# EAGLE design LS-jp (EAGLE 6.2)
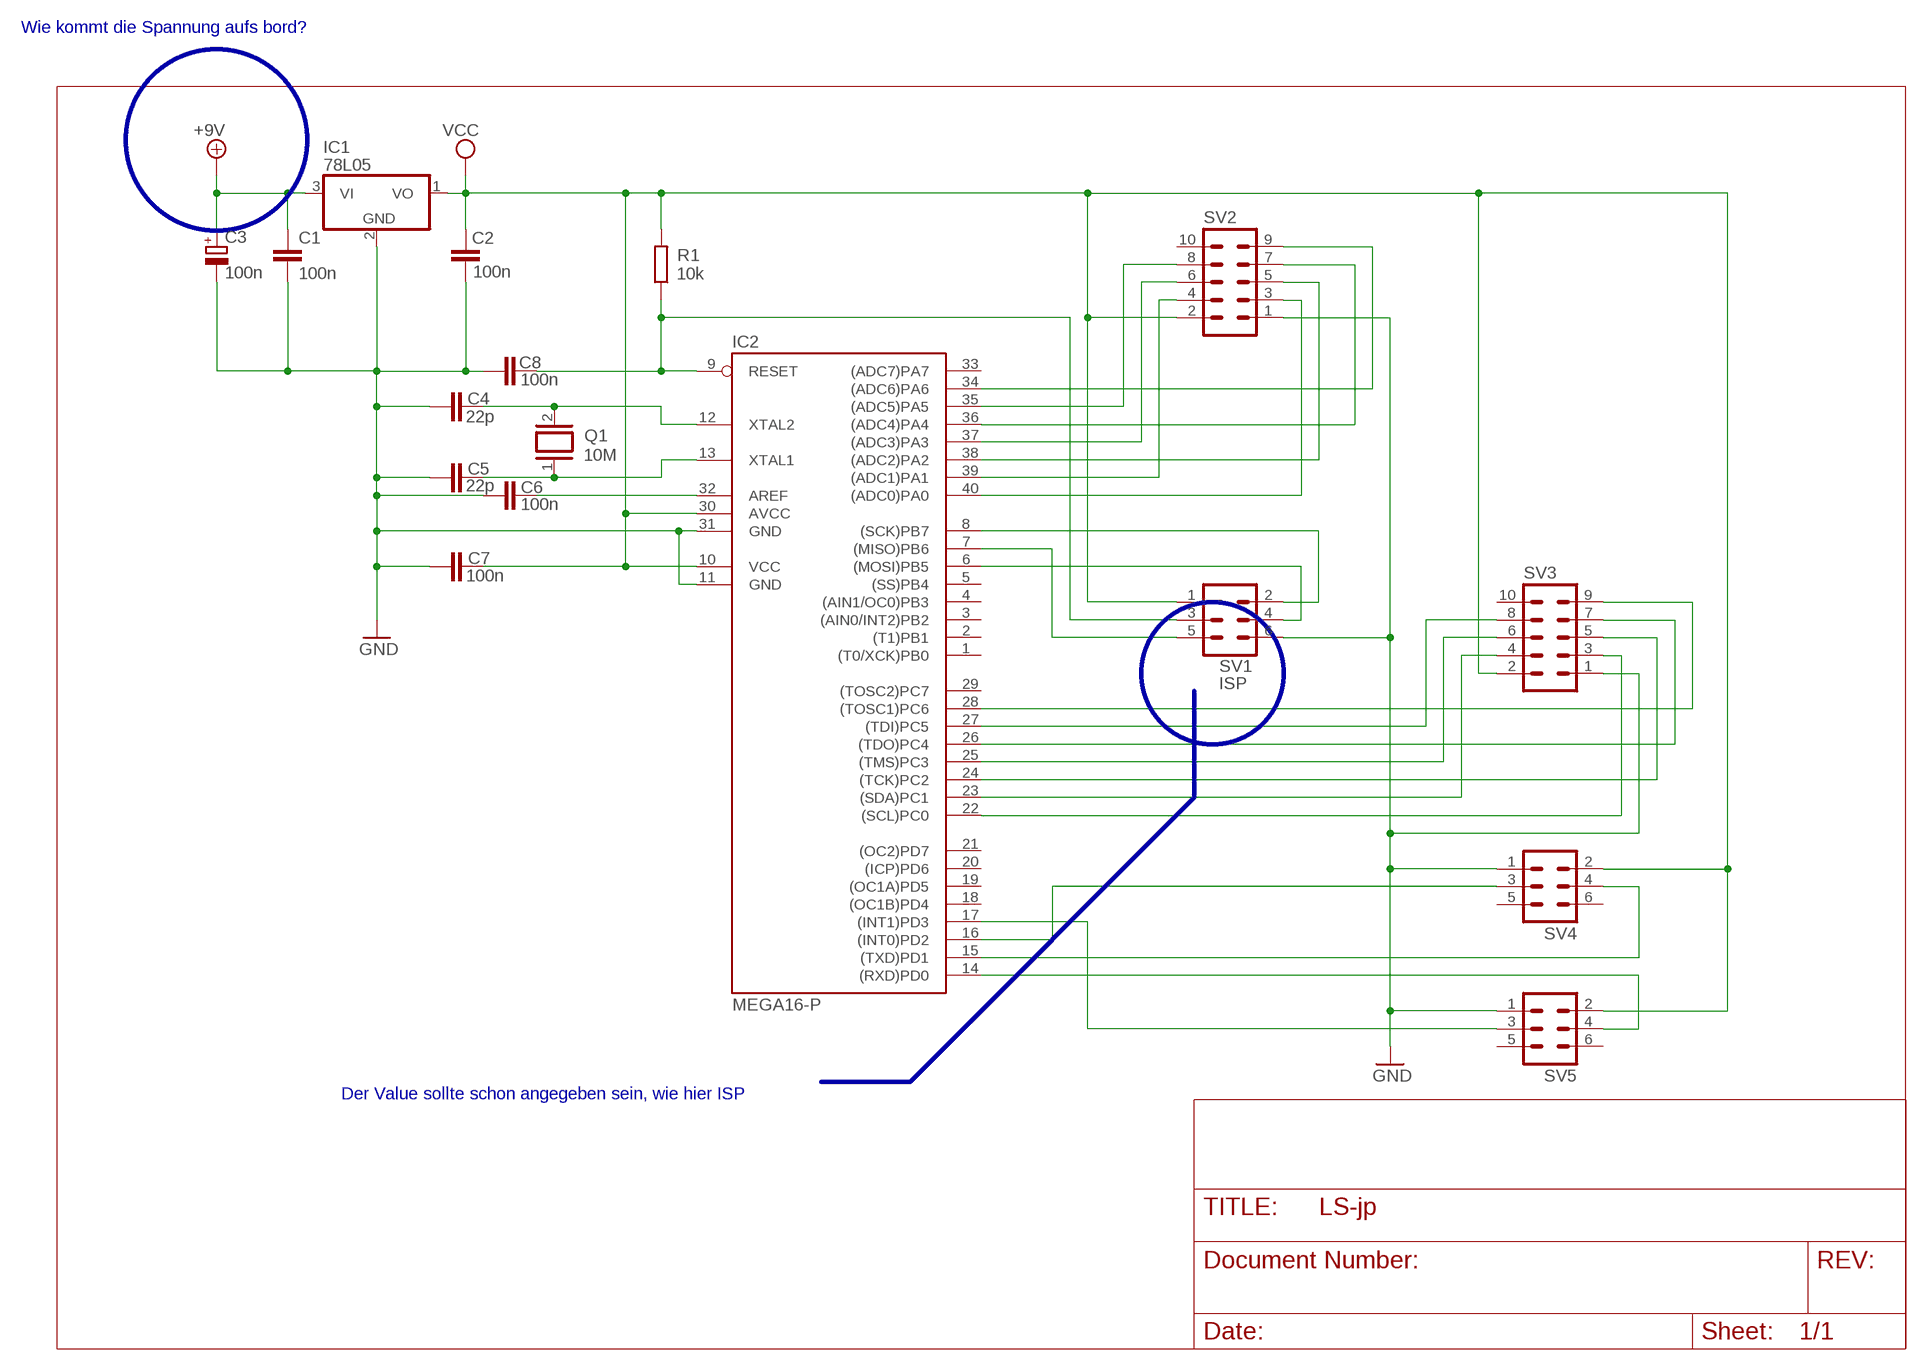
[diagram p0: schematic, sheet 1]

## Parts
C1  100n  C-EU025-024X044  [C025-024X044]
C2  100n  C-EU025-024X044  [C025-024X044]
C3  100n  CPOL-EUE2.5-7  [E2,5-7]
C4  22p  C-EU025-024X044  [C025-024X044]
C5  22p  C-EU025-024X044  [C025-024X044]
C6  100n  C-EU025-024X044  [C025-024X044]
C7  100n  C-EU025-024X044  [C025-024X044]
C8  100n  C-EU025-024X044  [C025-024X044]
IC1  78L05  78L12Z  [TO92]
IC2  MEGA16-P  [DIL40]
Q1  10M  XTAL/S  [QS]
R1  10k  R-EU_0207/10  [0207/10]
SV1  ISP  ML6  [ML6]
SV2  ML10  [ML10]
SV3  ML10  [ML10]
SV4  ML6  [ML6]
SV5  ML6  [ML6]

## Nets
+9V: C1.1 C3.+ IC1.3(VI)
GND: C1.2 C2.2 C3.- C4.2 C5.2 C6.2 C7.1 C8.1 IC1.2(GND) IC2.11(GND) IC2.31(GND) SV1.6 SV2.1 SV3.1 SV4.1 SV5.1
N$1: C6.1 IC2.32(AREF)
N$2: IC2.22((SCL)PC0) SV3.3
N$3: IC2.23((SDA)PC1) SV3.4
N$4: C8.2 IC2.9(RESET) R1.1 SV1.3
N$5: IC2.24((TCK)PC2) SV3.5
N$6: IC2.7((MISO)PB6) SV1.5
N$7: IC2.6((MOSI)PB5) SV1.4
N$8: C4.1 IC2.12(XTAL2) Q1.2
N$9: C5.1 IC2.13(XTAL1) Q1.1
N$10: IC2.8((SCK)PB7) SV1.2
N$11: IC2.40((ADC0)PA0) SV2.3
N$13: IC2.39((ADC1)PA1) SV2.4
N$14: IC2.25((TMS)PC3) SV3.6
N$15: IC2.38((ADC2)PA2) SV2.5
N$16: IC2.37((ADC3)PA3) SV2.6
N$17: IC2.36((ADC4)PA4) SV2.7
N$18: IC2.35((ADC5)PA5) SV2.8
N$19: IC2.26((TDO)PC4) SV3.7
N$20: IC2.27((TDI)PC5) SV3.8
N$21: IC2.28((TOSC1)PC6) SV3.9
N$22: IC2.34((ADC6)PA6) SV2.9
N$23: IC2.15((TXD)PD1) SV4.4
N$24: IC2.14((RXD)PD0) SV5.4
N$25: IC2.16((INT0)PD2) SV4.3
N$26: IC2.17((INT1)PD3) SV5.3
VCC: C2.1 C7.2 IC1.1(VO) IC2.10(VCC) IC2.30(AVCC) R1.2 SV1.1 SV2.2 SV3.2 SV4.2 SV5.2
Unconnected: IC2.1((T0/XCK)PB0) IC2.2((T1)PB1) IC2.3((AIN0/INT2)PB2) IC2.4((AIN1/OC0)PB3) IC2.5((SS)PB4) IC2.18((OC1B)PD4) IC2.19((OC1A)PD5) IC2.20((ICP)PD6) IC2.21((OC2)PD7) IC2.29((TOSC2)PC7) IC2.33((ADC7)PA7) SV2.10 SV3.10 SV4.5 SV4.6 SV5.5 SV5.6

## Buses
B$1

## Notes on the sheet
- Wie kommt die Spannung aufs bord?
- Der Value sollte schon angegeben sein, wie hier ISP

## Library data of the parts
C1 C2 C4-C8 = rcl:C-EU: CAPACITOR, European symbol
C3 = rcl:CPOL-EU: POLARIZED CAPACITOR, European symbol
IC1 = linear:78*: Positive VOLTAGE REGULATOR Source: http://cache.national.com/ds/LM/LM78L05.pdf http://www.fairchildsemi.com/ds/LM/LM7805.pdf
IC2 = atmel:MEGA16-P: MICROCONTROLLER 16 Kbytes FLASH 1 kbytes SRAM 512 bytes EEPROM USART 8-channel 10 bit ADC Source: avr.lbr; MPN: ATMEGA16-16PU; OC_FARNELL: 9171142; OC_NEWARK: 01M6885
Q1 = special:XTAL/S: CRYSTAL
R1 = rcl:R-EU_: RESISTOR, European symbol
SV1 SV4 SV5 = con-harting-ml:ML6: HARTING; OC_FARNELL: unknown; OC_NEWARK: unknown
SV2 SV3 = con-harting-ml:ML10: HARTING; OC_FARNELL: unknown; OC_NEWARK: unknown

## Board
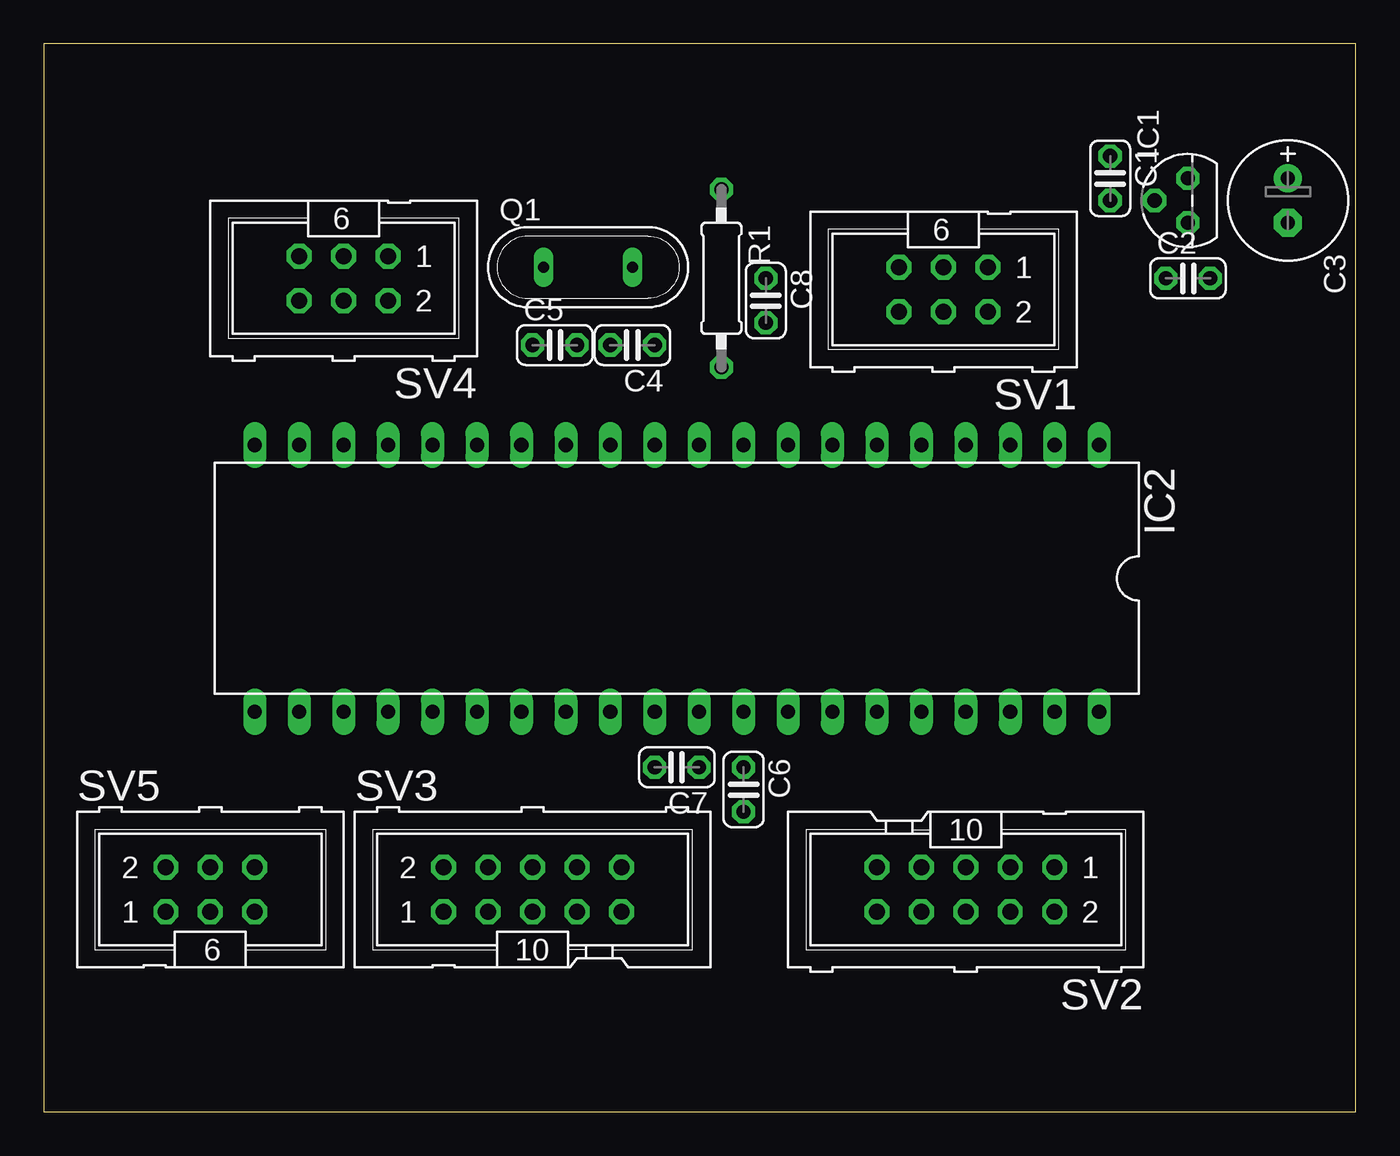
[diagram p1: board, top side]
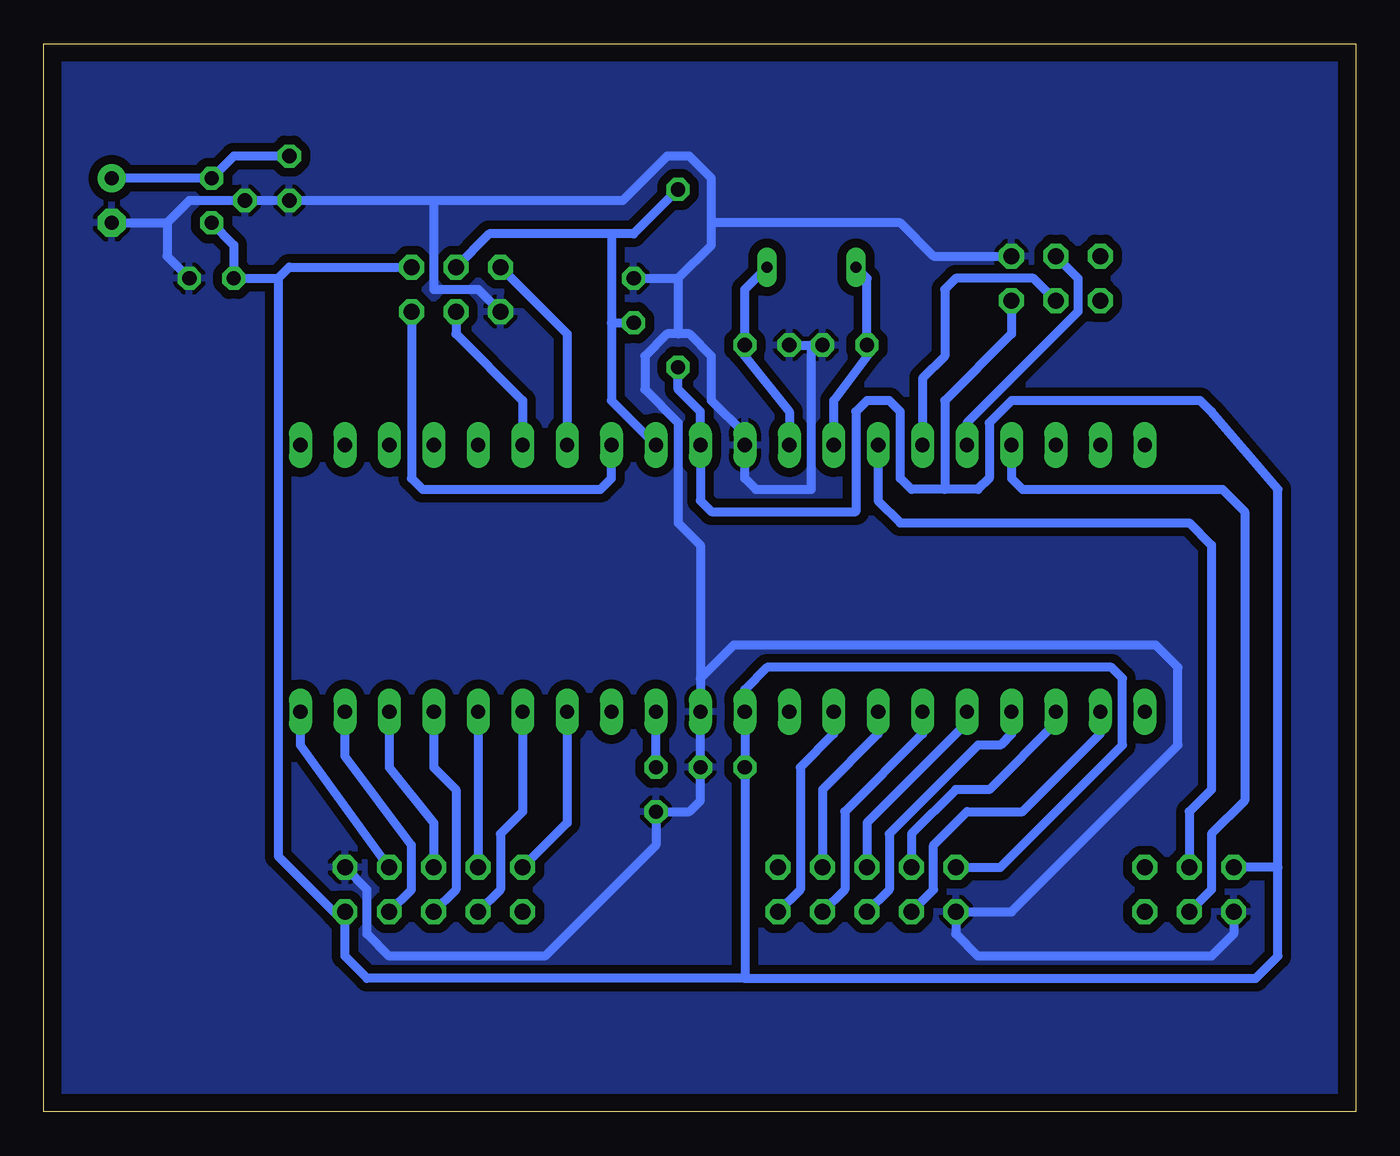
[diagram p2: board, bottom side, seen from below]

Size 75 x 61.03 mm. Coordinates in mm from the lower left corner, seen from the top.
Outline: 0,0 75,0 75,61.03 0,61.03 0,0
Copper layers (1*16): Top 0.035mm / dielectric 1.5mm / Bottom 0.035mm
Design rules "default": minimum track width 10mil, minimum drill 24mil, track to track 8mil, track to pad 8mil, pad to pad 8mil, via to via 8mil, smd to smd 8mil, copper to edge 40mil, drill to drill 8mil, minimum pad ring 10mil, minimum via ring 8mil, stop-mask expansion 4mil, vias tented up to drill 0mil, thermal gap 10mil

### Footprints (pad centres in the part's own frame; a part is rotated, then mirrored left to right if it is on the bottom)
C025-024X044 = drill 0.813 octagon: 1 -1.27,0; 2 1.27,0
E2,5-7 = drill 0.813 pad 1.6: + -1.27,0 | drill 0.813 pad 1.6 octagon: - 1.27,0
TO92 = drill 0.813 octagon: 1 -1.27,0; 2 0,1.905; 3 1.27,0
DIL40 = drill 0.813 long: 1 -24.13,-7.62; 2 -21.59,-7.62; 3 -19.05,-7.62; 4 -16.51,-7.62; 5 -13.97,-7.62; 6 -11.43,-7.62; 7 -8.89,-7.62; 8 -6.35,-7.62; 9 -3.81,-7.62; 10 -1.27,-7.62; 11 1.27,-7.62; 12 3.81,-7.62; 13 6.35,-7.62; 14 8.89,-7.62; 15 11.43,-7.62; 16 13.97,-7.62; 17 16.51,-7.62; 18 19.05,-7.62; 19 21.59,-7.62; 20 24.13,-7.62; 21 24.13,7.62; 22 21.59,7.62; 23 19.05,7.62; 24 16.51,7.62; 25 13.97,7.62; 26 11.43,7.62; 27 8.89,7.62; 28 6.35,7.62; 29 3.81,7.62; 30 1.27,7.62; 31 -1.27,7.62; 32 -3.81,7.62; 33 -6.35,7.62; 34 -8.89,7.62; 35 -11.43,7.62; 36 -13.97,7.62; 37 -16.51,7.62; 38 -19.05,7.62; 39 -21.59,7.62; 40 -24.13,7.62
QS = drill 0.61 long: 1 -2.54,0; 2 2.54,0
0207/10 = drill 0.813 octagon: 1 -5.08,0; 2 5.08,0
ML6 = drill 0.914 octagon: 1 -2.54,-1.27; 2 -2.54,1.27; 3 0,-1.27; 4 0,1.27; 5 2.54,-1.27; 6 2.54,1.27
ML10 = drill 0.914 octagon: 1 -5.08,-1.27; 2 -5.08,1.27; 3 -2.54,-1.27; 4 -2.54,1.27; 5 0,-1.27; 6 0,1.27; 7 2.54,-1.27; 8 2.54,1.27; 9 5.08,-1.27; 10 5.08,1.27

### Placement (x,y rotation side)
C1  60.96,53.34 270 top
C2  65.41,47.62 0 top
C3  71.12,52.07 270 top
C4  33.66,43.81 180 top
C5  29.21,43.81 0 top
C6  40.01,18.41 270 top
C7  36.2,19.68 180 top
C8  41.27,46.35 270 top
IC1  65.41,52.07 90 top
IC2  36.2,30.48 180 top
Q1  31.11,48.26 0 top
R1  38.73,47.62 270 top
SV1  51.44,46.99 180 top
SV2  52.7,12.7 180 top
SV3  27.94,12.7 0 top
SV4  17.14,47.62 180 top
SV5  9.53,12.7 0 top

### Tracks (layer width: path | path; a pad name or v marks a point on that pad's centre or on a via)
+9V
  Bottom 0.508: C1.1 64.14,54.61 IC1.3 C3.+
GND
  Bottom 0.508: 31.11,43.81 31.11,35.56 34.29,35.56 34.92,36.2 IC2.11 34.92,38.73 36.83,40.64 36.83,43.18 38.1,44.45 38.73,44.45 | SV4.1 24.13,48.89 26.04,50.8 36.83,50.8 | 38.73,47.62 36.83,49.53 36.83,50.8 | 36.83,50.8 36.83,53.34 38.1,54.61 39.37,54.61 41.91,52.07 52.7,52.07 | 52.7,52.07 52.7,46.99 50.16,46.99 SV1.6 | SV2.1 56.52,12.7 56.52,10.16 55.24,8.89 46.35,8.89 40.01,15.24 C6.2 38.1,17.14 37.47,17.78 C7.1 IC2.31 37.47,24.77 | C5.2 31.11,43.81 | C4.2 31.11,43.81 | 38.73,44.45 39.37,44.45 40.64,43.18 40.64,41.27 38.73,39.37 38.73,33.66 37.47,32.38 37.47,24.77 | C8.1 38.73,47.62 | 38.73,47.62 38.73,44.45 | 52.7,52.07 IC1.2 66.67,52.07 67.94,50.8 | 67.94,50.8 67.94,48.89 C2.2 | C3.- 67.94,50.8 | SV5.1 6.99,10.16 8.26,8.89 21.59,8.89 22.86,10.16 SV3.1 19.68,11.43 10.16,20.95 10.16,25.4 11.43,26.67 35.56,26.67 37.47,24.77
  pour Bottom (isolate 0.508): -3.81,-3.81 -3.81,64.77 80.01,64.77 80.01,30.48 80.01,-6.35 -3.81,-6.35
N$1
  Bottom 0.508: C6.1 IC2.32
N$2
  Bottom 0.508: IC2.22 14.61,21.59 19.05,17.14 22.23,17.14 24.13,15.24 24.13,12.7 SV3.3
N$3
  Bottom 0.508: IC2.23 17.14,22.22 20.95,18.41 22.86,18.41 25.4,15.88 SV3.4
N$4
  Bottom 0.508: IC2.9 42.55,40.64 42.55,45.09 | 42.55,50.16 41.27,50.16 R1.1 | 42.55,50.16 42.55,45.09 | 42.55,45.09 C8.2 | SV1.3 49.53,50.16 42.55,50.16
N$5
  Bottom 0.508: IC2.24 19.68,21.59 20.32,20.95 21.59,20.95 26.67,15.88 26.67,12.7 SV3.5
N$6
  Bottom 0.508: IC2.7 45.09,44.45 SV1.5
N$7
  Bottom 0.508: IC2.6 47.62,40.64 51.44,44.45 SV1.4
N$8
  Bottom 0.508: Q1.2 34.92,46.99 C4.1 34.92,43.18 32.38,40.01 IC2.12
N$9
  Bottom 0.508: IC2.13 29.84,40.64 27.94,43.18 C5.1 27.94,47.62 Q1.1
N$10
  Bottom 0.508: IC2.8 42.55,36.2 43.18,35.56 53.34,35.56 53.98,36.2 SV1.2
N$11
  Bottom 0.508: SV2.3 60.33,20.95 IC2.40
N$13
  Bottom 0.508: SV2.4 53.98,12.7 53.98,15.24 57.78,20.32 IC2.39
N$14
  Bottom 0.508: IC2.25 22.23,22.22 27.94,16.51 SV3.6
N$15
  Bottom 0.508: IC2.38 55.24,19.68 52.7,16.51 SV2.5
N$16
  Bottom 0.508: IC2.37 52.7,19.68 51.44,18.41 51.44,12.7 SV2.6
N$17
  Bottom 0.508: IC2.36 SV2.7
N$18
  Bottom 0.508: IC2.35 47.62,17.14 48.9,15.88 48.9,12.7 SV2.8
N$19
  Bottom 0.508: IC2.26 24.77,21.59 29.21,17.14 29.21,12.7 SV3.7
N$20
  Bottom 0.508: IC2.27 27.3,21.59 30.48,18.41 SV3.8
N$21
  Bottom 0.508: IC2.28 29.84,21.59 31.75,19.68 31.75,12.7 SV3.9
N$22
  Bottom 0.508: IC2.34 45.09,16.51 SV2.9
N$23
  Bottom 0.508: IC2.15 24.77,41.91 23.5,43.18 23.5,46.99 22.86,47.62 18.41,47.62 SV4.4
N$24
  Bottom 0.508: IC2.14 27.3,34.92 26.04,33.66 9.53,33.66 8.26,32.38 8.26,18.41 9.53,17.14 SV5.4
N$25
  Bottom 0.508: IC2.16 22.23,39.37 15.88,45.72 15.88,47.62 SV4.3
N$26
  Bottom 0.508: IC2.17 19.68,36.2 19.05,35.56 7.62,35.56 6.35,34.29 6.35,17.78 8.26,15.88 8.26,12.7 SV5.3
VCC
  Bottom 0.508: 4.45,13.97 4.45,35.56 8.26,40.01 8.89,40.64 19.68,40.64 20.95,39.37 20.95,36.2 21.59,35.56 23.5,35.56 | 34.92,7.62 56.52,7.62 57.78,8.89 SV2.2 58.42,11.43 61.59,14.61 61.59,47.62 | 34.92,7.62 C7.2 IC2.30 34.92,24.13 33.66,25.4 13.97,25.4 13.34,24.77 13.34,20.95 20.32,13.97 SV3.2 | R1.2 38.73,41.27 37.47,40.01 IC2.10 37.47,34.92 36.83,34.29 28.57,34.29 28.57,40.01 27.94,40.64 26.67,40.64 26.04,40.01 26.04,36.2 25.4,35.56 23.5,35.56 | 61.59,47.62 60.96,48.26 SV1.1 | IC1.1 64.14,49.53 C2.1 61.59,47.62 | SV4.2 19.68,44.45 23.5,40.64 23.5,35.56 | 34.92,7.62 5.71,7.62 4.45,8.89 4.45,13.97 | 4.45,13.97 SV5.2

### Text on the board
tRestrict: LS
